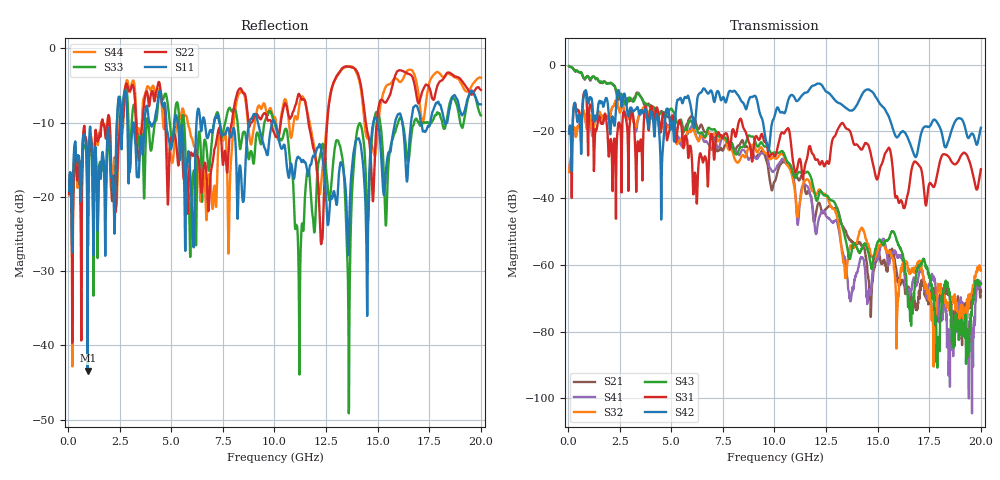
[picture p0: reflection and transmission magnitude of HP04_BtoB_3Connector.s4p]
# MHz S MA R 50.00
! FREQ  S11  S12  S13  S14
!  S21  S22  S23  S24
!  S31  S32  S33  S34
!  S41  S42  S43  S44
!  MAG  ANG  MAG  ANG  MAG  ANG  MAG  ANG
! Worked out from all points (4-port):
!   1996 points, 50 MHz to 20 GHz, reference 50 ohm
!   strongest paths, dB at 50 MHz, 5.04 GHz, 10.03 GHz, 15.02 GHz, 20 GHz:
!     S42: -20.6, -17.2, -14.8, -10.9, -18.9
!     S31: -20.6, -15.4, -27.5, -33.7, -31.4
!     S43: -0.5, -13.5, -26.4, -53.1, -65.6
!     S32: -32.1, -18.2, -28.2, -55.1, -61.7
!     S41: -32.2, -17.6, -31.5, -57.9, -65.7
!     S21: -0.5, -16.9, -34.9, -56.0, -67.9
!   lowest |S11| = -43.4 dB at 950 MHz (marker M1), VSWR 1.01, Z = 50.3 + j0.601 ohm
!   |S11| at or under -10 dB: start of sweep to 2.363 GHz; 7.338 GHz to 8.778 GHz (1.44 GHz wide, 17.9 % of centre); 10.02 GHz to 14.79 GHz (4.771 GHz wide, 38.5 % of centre)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
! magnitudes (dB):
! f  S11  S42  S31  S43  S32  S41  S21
! 50 MHz  -19.2  -20.6  -20.6  -0.5  -32.1  -32.2  -0.5
! 950 MHz  -43.4  -11.4  -21.4  -3.6  -18.6  -18.0  -3.4
! 10.37 GHz  -13.5  -14.2  -20.3  -25.9  -26.7  -28.3  -29.2
! 12.28 GHz  -14.0  -6.1  -29.1  -38.1  -38.3  -44.1  -43.7
! 13.67 GHz  -19.4  -13.8  -20.1  -58.0  -54.3  -70.1  -52.5
! 17.7 GHz  -8.3  -16.6  -36.7  -69.2  -86.0  -63.4  -68.3
! 20 GHz  -7.6  -18.9  -31.4  -65.6  -61.7  -65.7  -67.9
